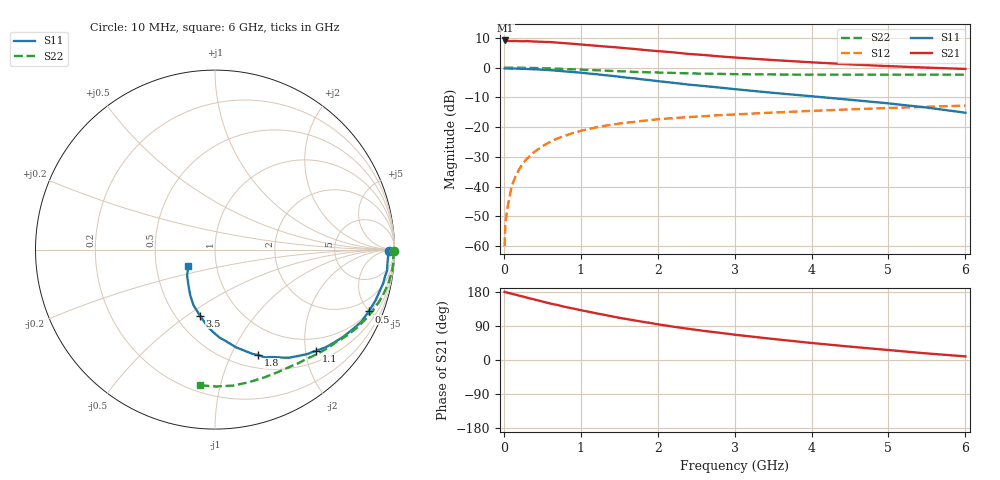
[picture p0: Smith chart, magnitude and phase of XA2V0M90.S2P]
! SIEMENS Discrete & RF Semiconductors
! BFY180
! Si NPN RF Bipolar Junction Transistor in MICRO-X
! VCE = 2 V  IC = 0.9 mA
! Common Emitter S-Parameters:  May  1997
# GHz  S  MA  R  50
!  f  S11  S21  S12  S22
! GHz  MAG  ANG  MAG  ANG  MAG  ANG  MAG  ANG
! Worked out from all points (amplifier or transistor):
!   36 points, 10 MHz to 6 GHz, reference 50 ohm
!   highest |S21| = 9.1 dB at 20 MHz (marker M1)
!   |S21| within 3 dB of that: start of sweep to 1.753 GHz
!   unconditionally stable (mu >= 1): 3.801 GHz to end of sweep
!   at 250 MHz: K = 0.08, MSG = 20.5 dB, |S12| = -32.1 dB
!   at 1.4 GHz: K = 0.50, MSG = 13.1 dB, |S12| = -19.2 dB
!   at 6 GHz: K = 1.06, MAG = 4.6 dB, |S12| = -12.8 dB
!   S11 on the Smith chart (normalised r, x): 10 MHz: 57, -12; 500 MHz: 1.06, -4.95; 1.1 GHz: 0.72, -2.22; 1.8 GHz: 0.65, -1.27; 3.5 GHz: 0.65, -0.56; 6 GHz: 0.73, -0.14
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0.01  0.9669 -0.4  2.791 179.7  0.001 86.5  0.9987 -0.3
0.02  0.9654 -0.9  2.862 178.8  0.0025 82.3  0.9999 -0.6
0.05  0.9654 -2.0  2.8 177.6  0.0046 87.3  0.9978 -1.3
0.1  0.9638 -4.5  2.801 175.0  0.01 88.3  0.9939 -2.7
0.15  0.966 -7.0  2.816 172.4  0.0146 85.2  0.9972 -4.0
0.2  0.9594 -8.8  2.778 169.8  0.0197 84.0  0.9944 -5.3
0.3  0.9491 -13.2  2.792 164.5  0.0295 80.5  0.9899 -7.9
0.5  0.9232 -21.9  2.716 154.4  0.0476 74.7  0.977 -13.0
0.6  0.9089 -26.3  2.688 149.1  0.0565 71.6  0.9691 -15.4
0.8  0.8633 -34.3  2.571 139.9  0.0721 65.9  0.9467 -20.2
1.1  0.7965 -45.0  2.388 127.5  0.0929 58.3  0.9137 -26.5
1.3  0.7502 -52.3  2.275 119.4  0.1048 53.8  0.8912 -30.6
1.5  0.7035 -58.7  2.173 111.3  0.1148 49.8  0.8696 -34.2
1.8  0.6345 -67.8  1.997 101.0  0.1274 45.2  0.8419 -39.2
2.2  0.5566 -77.9  1.808 88.0  0.1418 39.2  0.8146 -45.4
2.6  0.4912 -87.0  1.632 76.8  0.1528 34.9  0.7916 -50.9
3  0.4351 -95.0  1.48 66.8  0.1633 30.8  0.7775 -56.2
3.5  0.3771 -102.9  1.341 55.5  0.1758 26.7  0.7675 -62.5
4  0.3307 -111.5  1.228 44.9  0.1877 22.6  0.7632 -68.9
4.5  0.2886 -118.6  1.135 35.3  0.1991 18.7  0.7628 -75.6
5.5  0.2132 -136.7  1.001 17.3  0.2199 10.8  0.7631 -89.5
6  0.1748 -148.6  0.951 9.5  0.2301 6.5  0.7604 -96.5
